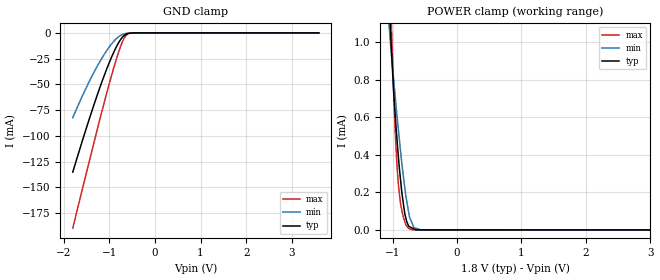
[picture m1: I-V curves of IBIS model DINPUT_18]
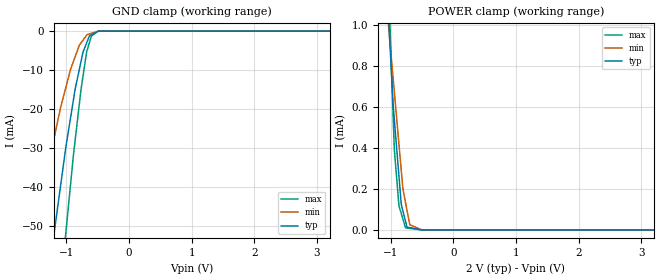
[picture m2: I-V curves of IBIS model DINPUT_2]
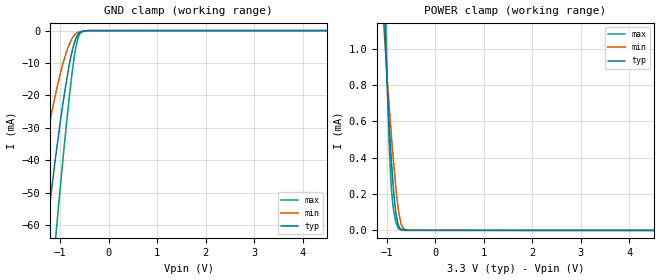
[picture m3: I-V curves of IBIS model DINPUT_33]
|Texas Instruments Incorporated
|Low-Power, 2/8-Channel, 24-Bit Analog Front-End for Biopotential Measurements
| Marketing part#  Digital I/O Voltage Range   Package-type   #pins
|ADS131E06IPAG   1.65V to 3.6 V   PQFP   64
|ADS131E06IPAGR   1.65V to 3.6 V   PQFP   64
[IBIS Ver]   4.0
[File name]   ads131e06.ibs
[File Rev]   1.0
[Date]   06/22/2012
[Source]   Texas Instruments Incorporated.
   Analog-eLab, HPA
   12500 TI Blvd
   Dallas, TX -75243
   For Support e-mail: elab_ibis@list.ti.com
[Notes]   Revision History:
   1.0: 06/22/2012 Initial Release
   - Pullup data is non-monotonic for CLK_2,DIO_2,DOUTRI_2
   and reflects circuit behavior
[Disclaimer]
 This product is designed as an aid for customers of Texas Instruments.
 No warranties, either expressed or implied, with respect to this third
 party software (if any) or with respect to its fitness for any
 particular purpose is claimed by Texas Instruments or the author. The
 software (if any) is provided solely on an "as is" basis. The entire
 risk as to its quality and performance is with the customer
[Copyright] (C) Copyright 2012 Texas Instruments Incorporated.
   All rights reserved.
|   ADS131E06
[Component]   ads131e06pag
[Manufacturer] TI
[Package]   |PAG (PQFP) - 64 pin
| variable   typ   min   max
R_pkg  0.007601   0.007601   0.007601
L_pkg  1.950031nH 1.950031nH 1.950031nH
C_pkg  0.403260pF 0.403260pF 0.403260pF
[Pin] signal_name   model_name   R_pin   L_pin   C_pin
1   NC   NC   0.00802  2.18050nH  0.36893pF
2   NC   NC   0.00796  2.08284nH  0.44422pF
3   NC   NC   0.00774  2.00579nH  0.43874pF
4   NC   NC   0.00761  1.96075nH  0.41947pF
5   IN6N   TERM   0.00767  1.93366nH  0.41193pF
6   IN6P   TERM   0.00745  1.86807nH  0.39172pF
7   IN5N   TERM   0.00723  1.80701nH  0.38069pF
8   IN5P   TERM   0.00717  1.80128nH  0.34665pF
9   IN4N   TERM   0.00717  1.80167nH  0.34655pF
10   IN4P   TERM   0.00723  1.80708nH  0.38064pF
11   IN3N   TERM   0.00746  1.86875nH  0.39156pF
12   IN3P   TERM   0.00767  1.93382nH  0.41197pF
13   IN2N   TERM   0.00762  1.96069nH  0.41976pF
14   IN2P   TERM   0.00774  2.00536nH  0.43931pF
15   IN1N   TERM   0.00796  2.08200nH  0.44472pF
16   IN1P   TERM   0.00802  2.18040nH  0.36892pF
17   TESTP_PACE_OUT1   TERM   0.00802  2.18050nH  0.36893pF
18   TESTP_PACE_OUT2   TERM   0.00796  2.08284nH  0.44422pF
19   AVDD   POWER   0.00774  2.00579nH  0.43874pF
20   AVSS   GND   0.00761  1.96075nH  0.41948pF
21   AVDD   POWER   0.00767  1.93365nH  0.41193pF
22   AVDD   POWER   0.00745  1.86807nH  0.39171pF
23   AVSS   GND   0.00723  1.80701nH  0.38069pF
24   VREFP   TERM   0.00717  1.80128nH  0.34665pF
25   VREFN   TERM   0.00717  1.80166nH  0.34656pF
26   VCAP4   TERM   0.00723  1.80707nH  0.38065pF
27   NC   NC   0.00746  1.86875nH  0.39156pF
28   VCAP1   TERM   0.00767  1.93381nH  0.41197pF
29   NC   NC   0.00762  1.96066nH  0.41979pF
30   VCAP2   TERM   0.00774  2.00511nH  0.43938pF
31   RESV1   DINPUT  0.00796  2.08195nH  0.44475pF
32   AVSS   GND   0.00802  2.18014nH  0.36899pF
33   DGND   GND   0.00802  2.18049nH  0.36893pF
34   DIN   DINPUT  0.00796  2.08283nH  0.44422pF
35   _PWDN   DINPUT  0.00774  2.00579nH  0.43874pF
36   _RESET   DINPUT  0.00761  1.96075nH  0.41947pF
37   CLK   CLK   0.00767  1.93366nH  0.41193pF
38   START   DINPUT  0.00745  1.86807nH  0.39172pF
39   _CS   DINPUT  0.00723  1.80701nH  0.38069pF
40   SCLK   DIO   0.00717  1.80128nH  0.34665pF
41   DAISY_IN   DIO   0.00717  1.80167nH  0.34655pF
42   GPIO1   DIO   0.00723  1.80708nH  0.38064pF
43   DOUT   DOUTRI  0.00746  1.86875nH  0.39156pF
44   GPIO2   DIO   0.00767  1.93382nH  0.41197pF
45   GPIO3   DIO   0.00762  1.96069nH  0.41976pF
46   GPIO4   DIO   0.00774  2.00536nH  0.43931pF
47   _DRDY   DOUTRI  0.00796  2.08200nH  0.44472pF
48   DVDD   POWER   0.00802  2.18040nH  0.36892pF
49   DGND   GND   0.00802  2.18051nH  0.36893pF
50   DVDD   POWER   0.00796  2.08284nH  0.44422pF
51   DGND   GND   0.00774  2.00579nH  0.43874pF
52   CLKSEL   DINPUT  0.00761  1.96073nH  0.41948pF
53   AVSS1   GND   0.00767  1.93366nH  0.41193pF
54   AVDD1   POWER   0.00745  1.86807nH  0.39171pF
55   VCAP3   TERM   0.00723  1.80701nH  0.38069pF
56   AVDD   POWER   0.00717  1.80128nH  0.34665pF
57   AVSS   GND   0.00717  1.80166nH  0.34656pF
58   AVSS   GND   0.00723  1.80707nH  0.38065pF
59   AVDD   POWER   0.00746  1.86875nH  0.39156pF
60   OPAMPP   TERM   0.00767  1.93381nH  0.41197pF
61   OPAMPN   TERM   0.00762  1.96066nH  0.41979pF
62   NC   NC   0.00774  2.00511nH  0.43938pF
63   OPAMPOUT   TERM   0.00796  2.08195nH  0.44475pF
64   NC   NC   0.00802  2.18014nH  0.36899pF
[Model Selector]  DINPUT
DINPUT_18  1.8V digital input
DINPUT_2   2.0V digital input
DINPUT_33  3.3V digital input
[Model Selector]  CLK
CLK_18  1.8V digital I/O
CLK_2   2.0V digital I/O
CLK_33  3.3V digital I/O
[Model Selector] DIO
DIO_18  1.8V digital I/O
DIO_2   2.0V digital I/O
DIO_33  3.3V digital I/O
[Model Selector]  DOUTRI
DOUTRI_18  1.8V digital I/O
DOUTRI_2   2.0V digital I/O
DOUTRI_33  3.3V digital I/O
[Model Selector]  TERM
TERM_18  1.8V digital I/O
TERM_2   2.0V digital I/O
TERM_33  3.3V digital I/O
|   TERM Model
[Model] TERM_18
Model_type Terminator
|for ADS1291, ADS1292, ADS1294, ADS1296, and ADS1298 products
C_comp   1e-20   1e-20   1e-20
| variable   typ   min   max
[Voltage Range]   1.8V   1.65V   2V
[POWER Clamp Reference]  1.8V   1.65V   2V
[GND Clamp Reference]   0.0V   0.0V   0.0V
|Operating Temperature
[Temperature Range]   27   85   -40
|   TERM Model
[Model] TERM_2
Model_type Terminator
|for ADS1299 products
C_comp   1e-20   1e-20   1e-20
| variable   typ   min   max
[Voltage Range]   2.0V   1.8V   2.2V
[POWER Clamp Reference]  2.0V   1.8V   2.2V
[GND Clamp Reference]   0.0V   0.0V   0.0V
|Operating Temperature
[Temperature Range]   27   85   -40
|   TERM Model
[Model] TERM_33
Model_type Terminator
|for all products
C_comp   1e-20   1e-20   1e-20
| variable   typ   min   max
[Voltage Range]   3.3V   3.0V   3.6V
[POWER Clamp Reference]  3.3V   3.0V   3.6V
[GND Clamp Reference]   0.0V   0.0V   0.0V
|Operating Temperature
[Temperature Range]   27   85   -40
| Models and submodels in the file (15): DINPUT_18 (Input), DINPUT_2 (Input), DINPUT_33 (Input), CLK_18 (I/O), CLK_2 (I/O), CLK_33 (I/O), DIO_18 (I/O), DIO_2 (I/O), DIO_33 (I/O), DOUTRI_18 (I/O), DOUTRI_2 (I/O), DOUTRI_33 (I/O), TERM_18 (Terminator), TERM_2 (Terminator), TERM_33 (Terminator)
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|   DINPUT 1.8V Model
[Model]   DINPUT_18
Model_type   Input
|for ADS1291, ADS1292, ADS1294, ADS1296, and ADS1298 products
|Signals   DIN, CLKSEL, START, _CS, _RESET, _PWDN, RESV1
Vinl = 0.36
Vinh = 1.44
|   typ   min   max
|   (nom PVT)   (Fast PVT)   (slow PVT)
|C_comp from frequency sweep method (F=64MHz)
|C_comp   2.5452470e-12   1.8682050e-12   3.0942680e-12
|C_comp from LC tank measurement(L=1nH)
C_comp   1.762E-12   1.432E-12   2.090E-12
| Where   nom PVT is  Nominal Process, 1.8V, 27C
|   Fast PVT is Strong Process, 2V, -40C
|   Slow PVT is Weak Process, 1.65V, 85C
[Voltage Range]   1.8   1.65   2
[Temperature Range]   27   85   -40
[Power Clamp Reference]   1.8   1.65   2
[GND Clamp Reference]   0   0   0
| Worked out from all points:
|   GND clamp passes 1 mA (typ) near -0.62 V on its own axis
|   POWER clamp passes 1 mA (typ) near -1.02 V on its own axis
[GND Clamp]
|   Voltage   I(typ)   I(min)   I(max)
-1.8V     -135.3mA   -82.39mA   -189.7mA
-1.616V   -108.7mA   -63.88mA   -156.7mA
-1.379V   -75.57mA   -41.98mA   -114.3mA
-1.23V    -56.14mA   -29.74mA   -88.13mA
-1.062V   -35.84mA   -17.66mA   -59.61mA
-932.5mV  -21.81mA   -9.837mA   -38.75mA
-792.7mV  -9.398mA   -3.624mA   -18.42mA
-709mV    -4.1mA     -1.551mA   -8.389mA
-674.7mV  -2.584mA   -992.8uA   -5.261mA
-611mV    -858.6uA   -415.2uA   -1.62mA
-440mV    -12.33uA   -13.16uA   -11.39uA
3.595V    0A         0A         0A
[POWER Clamp]
|   Voltage   I(typ)   I(min)   I(max)
-1.8V     10.43mA    8.127mA    13.16mA
-1.051V   1.214mA    1.076mA    1.506mA
-1.037V   1.102mA    1.014mA    1.323mA
-1.017V   953.2uA    928.3uA    1.088mA
-954.5mV  588uA      692.9uA    491.3uA
-907.1mV  378.3uA    524.9uA    231.9uA
-870.3mV  246.8uA    400.7uA    128.7uA
-813.8mV  94.97uA    234.6uA    48.61uA
-753.5mV  23.33uA    100.5uA    8.199uA
-670.2mV  5.85uA     13.5uA     989.7nA
-565.3mV  691.6nA    574.1nA    965.3nA
3.595V    0A         0A         0A
|   DINPUT 2.0V Model
[Model]   DINPUT_2
Model_type   Input
|for ADS1299 products
|Signals   DIN, CLKSEL, START, _CS, _RESET, _PWDN, RESV1
Vinl = 0.4
Vinh = 1.6
|   typ   min   max
|   (nom PVT)   (Fast PVT)   (slow PVT)
|C_comp from LC tank measurement(L=1nH)
C_comp   1.762E-12   1.413E-12   2.080E-12
| Where   nom PVT is  Nominal Process, 2V, 27C
|   Fast PVT is Strong Process, 2.2V, -40C
|   Slow PVT is Weak Process, 1.8V, 85C
[Voltage Range]   2   1.8   2.2
[Temperature Range]   27   85   -40
[Power Clamp Reference]   2   1.8   2.2
[GND Clamp Reference]   0   0   0
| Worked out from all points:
|   GND clamp passes 1 mA (typ) near -0.60 V on its own axis
|   POWER clamp passes 1 mA (typ) near -1.02 V on its own axis
[GND Clamp]
|   Voltage   I(typ)   I(min)   I(max)
-2V       -165mA     -103.7mA   -225.8mA
-1.501V   -92.94mA   -52.98mA   -136.6mA
-1.42V    -81.21mA   -45.88mA   -122mA
-1.201V   -52.44mA   -27.8mA    -83.48mA
-1.004V   -29.36mA   -14.21mA   -51.08mA
-893.3mV  -18.24mA   -8.053mA   -32.73mA
-766.2mV  -7.786mA   -3.015mA   -14.98mA
-732.1mV  -5.289mA   -2.272mA   -11.33mA
-669.4mV  -2.756mA   -907.9uA   -4.968mA
-600.8mV  -975.6uA   -568.8uA   -1.286mA
-469.4mV  -26.5uA    -23.94uA   -30.72uA
3.994V    0A         0A         0A
[POWER Clamp]
|   Voltage   I(typ)   I(min)   I(max)
-2V       13.12mA    10.41mA    16.44mA
-1.035V   1.096mA    1.005mA    1.318mA
-1.011V   911.5uA    919.2uA    1.019mA
-1.005V   876.1uA    898.5uA    953.1uA
-960.4mV  615.3uA    745.1uA    568.7uA
-939.7mV  537.9uA    673.3uA    391.2uA
-867.1mV  267.1uA    422uA      122.3uA
-827.1mV  122.7uA    283.5uA    78.12uA
-760.4mV  42.06uA    132.4uA    10.33uA
-693.7mV  11.43uA    25.58uA    7.717uA
-494.6mV  0A         53.96nA    0A
3.994V    0A         0A         0A
|   DINPUT 3.3V Model
[Model]   DINPUT_33
Model_type   Input
|for all products
|Signals   DIN, CLKSEL, START, _CS, _RESET, _PWDN, RESV1
Vinl = 0.66
Vinh = 2.64
|   typ   min   max
|   (nom PVT)   (Fast PVT)   (slow PVT)
|C_comp from frequency sweep method (F=64MHz)
|C_comp   2.2874600e-12   1.7279600e-12   2.8419150e-12
|C_comp from LC tank measurement(L=1nH)
C_comp   1.652E-12   1.343E-12   1.968E-12
| Where   nom PVT is  Nominal Process, 3.3V, 27C
|   Fast PVT is Strong Process, 3.6V, -40C
|   Slow PVT is Weak Process, 3V, 85C
[Voltage Range]   3.3   3   3.6
[Temperature Range]   27   85   -40
[Power Clamp Reference]   3.3   3   3.6
[GND Clamp Reference]   0   0   0
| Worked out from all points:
|   GND clamp passes 1 mA (typ) near -0.62 V on its own axis
|   POWER clamp passes 1 mA (typ) near -1.02 V on its own axis
[GND Clamp]
|   Voltage   I(typ)   I(min)   I(max)
-3.3V     -365.5mA   -258.9mA   -460.2mA
-1.597V   -106mA     -62.12mA   -153.3mA
-1.296V   -64.68mA   -35.02mA   -99.72mA
-1.202V   -52.57mA   -27.66mA   -83.32mA
-1.089V   -38.89mA   -19.5mA    -64.05mA
-1.054V   -34.94mA   -17.04mA   -58.12mA
-812mV    -10.83mA   -4.451mA   -21.03mA
-706.7mV  -3.936mA   -1.508mA   -8.155mA
-630.7mV  -1.241mA   -525.7uA   -2.473mA
-554.3mV  -267.8uA   -311.7uA   -396.5uA
-426.7mV  -11.62uA   -13.55uA   -7.153uA
6.59V     0A         0A         0A
[POWER Clamp]
|   Voltage   I(typ)   I(min)   I(max)
-3.3V     30.92mA    25.65mA    38.05mA
-1.057V   1.262mA    1.102mA    1.572mA
-1.022V   988.4uA    952.9uA    1.141mA
-1.015V   943.9uA    924uA      1.063mA
-972.9mV  681.5uA    762.7uA    640.3uA
-942.5mV  532.8uA    652.4uA    408.8uA
-901.3mV  364.2uA    503.2uA    211.4uA
-859.7mV  209.7uA    372.2uA    108.6uA
-812mV    91.53uA    228.1uA    43.91uA
-750.2mV  23.25uA    90.32uA    9.292uA
-689.4mV  5.727uA    26.05uA    923.4nA
6.59V     0A         0A         0A
